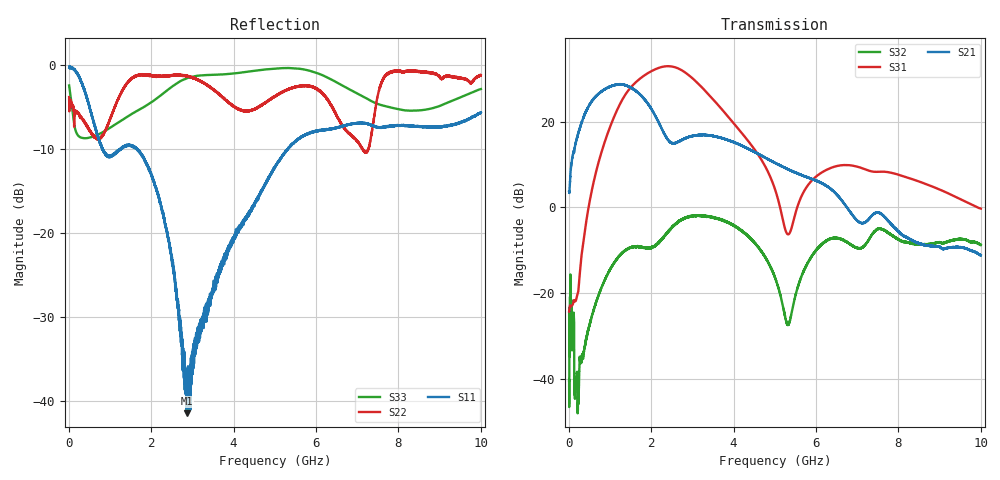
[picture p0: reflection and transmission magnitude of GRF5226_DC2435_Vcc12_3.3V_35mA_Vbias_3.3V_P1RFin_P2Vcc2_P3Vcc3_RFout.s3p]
!Keysight Technologies,N5245B,MY56052315,A.20.20.05
!Date: Friday, August 21, 2026 14:55:17
!Correction: S11(C  3-Port  )
!S12(C  3-Port  )
!S13(C  3-Port  )
!S21(C  3-Port  )
!S22(C  3-Port  )
!S23(C  3-Port  )
!S31(C  3-Port  )
!S32(C  3-Port  )
!S33(C  3-Port  )
!S3P File: Measurements: <S11,S12,S13>,
!<S21,S22,S23>,
!<S31,S32,S33>:
# Hz S  dB  R 50
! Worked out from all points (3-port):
!   9991 points, 10 MHz to 10 GHz, reference 50 ohm
!   strongest paths, dB at 10 MHz, 2.507 GHz, 5.005 GHz, 7.503 GHz, 10 GHz:
!     S21: 3.8, 15.0, 10.4, -1.2, -11.2
!     S31: -24.3, 32.9, 4.2, 8.3, -0.3
!     S32: -40.4, -4.6, -16.3, -5.0, -8.8
!   lowest |S11| = -41.4 dB at 2.873 GHz (marker M1), VSWR 1.02, Z = 50.8 + j0.202 ohm
!   |S11| at or under -10 dB: 819.5 MHz to 824.7 MHz (5.157 MHz wide, 0.627 % of centre); 825.2 MHz to 1.265 GHz (439.5 MHz wide, 42.1 % of centre); 1.651 GHz to 5.318 GHz (3.667 GHz wide, 105 % of centre)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
1e7  -0.38 -1.9  -58.42 -178.7  -51.88 -120.0
     3.75 59.9  -3.87 -40.1  -53.53 -136.2
     -24.33 -154.1  -40.42 57.5  -2.49 -54.1
4.77e8  -4.60 -76.1  -42.80 110.2  -65.46 69.2
        23.49 30.5  -7.53 172.3  -51.94 -38.6
        -0.26 9.4  -28.69 8.0  -8.72 -156.3
8.91e8  -10.64 -92.4  -38.92 77.7  -64.53 125.9
        27.70 -16.7  -7.82 -166.8  -40.17 -113.4
        15.79 -40.9  -16.66 -41.5  -7.86 -156.2
1.431e9  -9.58 -118.1  -37.81 83.0  -62.74 106.7
         28.34 -83.9  -2.16 -167.9  -33.71 179.2
         27.14 -122.5  -9.72 -103.2  -6.16 -155.3
1.956e9  -12.64 -175.0  -34.74 83.9  -59.14 66.7
         23.72 -142.5  -1.31 162.1  -32.26 131.9
         31.58 158.8  -9.38 -137.6  -4.65 -156.4
2.421e9  -20.87 135.8  -33.39 83.9  -57.61 90.5
         15.69 -153.5  -1.32 142.5  -30.62 109.2
         33.00 92.9  -5.53 -147.5  -2.94 -160.6
2.873e9  -41.45 13.6  -32.26 86.8  -55.41 83.4
         16.37 -141.8  -1.36 133.9  -28.73 79.0
         31.20 29.6  -2.31 174.3  -1.62 -172.0
3.499e9  -27.17 -138.7  -29.80 90.3  -54.93 68.1
         16.67 -171.0  -2.95 134.8  -28.84 39.9
         25.29 -37.1  -2.29 121.4  -1.22 172.3
5.005e9  -12.25 176.9  -26.59 73.9  -55.54 73.6
         10.42 122.1  -3.78 114.7  -36.99 -30.6
         4.25 -130.7  -16.34 29.2  -0.48 156.1
1e10  -5.70 110.5  -25.44 37.3  -52.22 26.6
      -11.19 54.3  -1.26 88.0  -30.59 -22.7
      -0.27 122.9  -8.81 -42.0  -2.91 76.9
